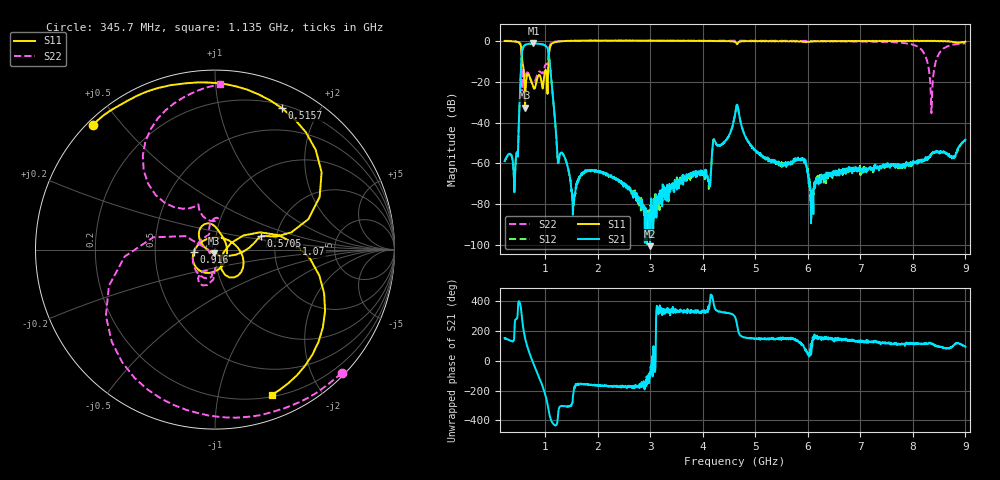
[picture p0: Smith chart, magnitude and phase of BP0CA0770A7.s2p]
!Agilent Technologies,E8358A,US41080443,A.07.50.56
!Agilent E8358A: A.07.50.56
!Date: Tuesday, April 11, 2017 15:48:33
!Correction: S11(Full 2 Port(1,2))
!S21(Full 2 Port(1,2))
!S12(Full 2 Port(1,2))
!S22(Full 2 Port(1,2))
!S2P File: Measurements: S11, S21, S12, S22:
# Hz S  dB  R 50
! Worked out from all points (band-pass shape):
!   1601 points, 225 MHz to 9 GHz, reference 50 ohm
!   highest |S21| = -1.28 dB at 773.4 MHz (marker M1); lowest = -100.5 dB at 2.995 GHz (marker M2)
!   |S21| within 3 dB of the highest: 564 MHz to 1.05 GHz (486.2 MHz wide, 60.2 % of centre)
!   lowest |S11| = -32.8 dB at 614.4 MHz (marker M3), VSWR 1.05, Z = 49.2 - j2.13 ohm
!   |S11| at or under -10 dB: 562.7 MHz to 1.062 GHz (498.9 MHz wide, 61.4 % of centre)
!   |S22| runs from -35.4 to 0.1 dB; largest |S21 - S12| = 0.01
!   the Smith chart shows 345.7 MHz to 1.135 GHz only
!   S11 on the Smith chart (normalised r, x): 345.7 MHz: 0.02, +0.42; 515.7 MHz: 0.24, +1.55; 570.5 MHz: 1.67, +0.27; 916 MHz: 0.79, -0.02; 1.07 GHz: 2.63, +0.19; 1.135 GHz: 0.22, -1.45
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2.25e8  -0.14 154.1  -58.83 152.4  -58.98 150.0  -0.04 -24.6
3.456562e8  -0.24 134.4  -55.75 134.1  -55.80 133.9  -0.12 -44.2
4.388906e8  -0.41 109.2  -57.84 -82.4  -57.78 -82.4  -0.36 -70.3
5.156719e8  -1.19 64.7  -26.41 28.0  -26.48 28.2  -1.47 -122.0
5.705156e8  -11.44 16.1  -3.66 -118.7  -3.74 -118.5  -15.57 -93.2
6.143906e8  -32.76 -109.8  -2.03 153.2  -2.12 153.3  -18.15 -108.7
7.734375e8  -22.82 39.1  -1.28 -18.5  -1.37 -18.4  -21.04 116.0
9.160312e8  -18.53 -174.3  -1.58 -140.9  -1.67 -140.7  -15.42 84.5
1.069594e9  -6.90 3.7  -7.24 15.6  -7.33 15.9  -4.51 131.9
1.135406e9  -1.22 -68.5  -24.84 -56.6  -24.87 -56.3  -0.72 88.3
1.245094e9  -0.47 -109.7  -59.86 2.7  -59.94 4.6  -0.31 59.6
1.519312e9  -0.06 -140.5  -78.95 76.8  -78.26 97.7  -0.08 32.0
1.689328e9  0.07 -150.1  -64.65 -155.4  -65.39 -157.0  -0.11 21.8
2.994609e9  0.07 -176.8  -100.47 -77.9  -92.30 -99.8  -0.09 -20.6
3.153656e9  -0.04 -178.4  -77.12 -3.7  -78.77 -36.3  0.01 -24.2
4.113422e9  -0.10 169.4  -69.17 -11.3  -72.53 2.6  -0.04 -41.6
4.6125e9  -0.53 159.7  -36.16 -66.5  -36.26 -66.9  -0.05 -50.0
5.917781e9  -0.47 140.7  -58.23 99.1  -57.93 96.9  -0.14 -71.4
6.076828e9  -0.39 139.1  -77.01 130.4  -82.69 101.2  -0.14 -74.1
7.541156e9  -0.18 118.5  -61.40 121.4  -60.74 121.0  -0.63 -127.4
8.352844e9  -0.05 108.1  -55.68 116.3  -55.27 116.8  -35.44 47.5
9e9  -0.41 104.7  -48.37 93.5  -48.68 94.3  -1.33 -143.9
